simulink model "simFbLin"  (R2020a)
settings: Solver=ode15s  StartTime=0.0  StopTime=tsim  MaxStep=1  RelTol=1e-3
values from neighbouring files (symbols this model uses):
  dQ2 = Q20+0    (= 836)    [runTransformations.m]
  dT0 = T00+0    (= 10)    [runTransformations.m]
  dv2 = v20+0    (= 0)    [runTransformations.m]    (also in FcOL.m = -0.391; runTransfOL.m = -1)
  nd = 2    [runTransformations.m]    (also in Main.m = size(d0,2); Main_OL.m = size(d0,2); runTestCalcBlk.m = size(d0,2); runTransf.m = size(d0,2))
  np = length(p)    [runTransformations.m]    (also in runH2Psim.m = length(param); Main.m = size(p,2); Main_OL.m = size(p,2); runTestCalcBlk.m = size(p,2))
  nu = 1    [runTransformations.m]    (also in runH2Psim.m = length(u0); Main.m; Main_OL.m; runTestCalcBlk.m)
  nx = 2    [runTransformations.m]    (also in H2P_Turbine_driven.m = param(end); runTD.m = length(x0); H2P_Boiler_driven.m = param(end); runBD.m = length(x0))
  p = [p;tau01;tau02]    [runTransformations.m]    (also in Main.m = [N, Fc0, rhoc, rhoh,U,A,cpc,cph]; Main_OL.m = [N, Fc0, rhoc, rhoh,U,A,cpc,cph]; runTestCalcBlk.m = [N, Fc0, rhoc, rhoh,U,A,cpc,cph]; NonlinearMap.m = [U;A;Fc(i);Fh;cpc;cph;Tcin;Thin])
  Q20 = -F*cp*(T10-T20)    (= 836)    [runTransformations.m]
  T00 = 10    [runTransformations.m]
  tdQ2 = 10    [runTransformations.m]
  tdT0 = 10    [runTransformations.m]
  tsp = 10    [runTransformations.m]
  v20 = 0    [runTransformations.m]    (also in runTransfOL.m = v00)
  x0 = [T10;T20]    [runTransformations.m]    (also in runTD.m = [TE0;TD0;TSh0;MD0; MSh0;w0;TA0;0;0;0;0;0;0;0;0;0]; runBD.m = [TE0;TD0;TSh0;MD0; MSh0;w0;TA0;0;0;0;0;0;0;0;0;0]; runFP.m = [TE0;TD0;TSh0;MD0; MSh0;w0;TA0;0;0;0;0;0;0;0]; runFPV2.m = [TE0;TD0;TSh0;MD0; MSh0;w0;TA0;0;0;0;0;0;0;0])
undefined symbols (not defined in the file or in its folder): TanksODE

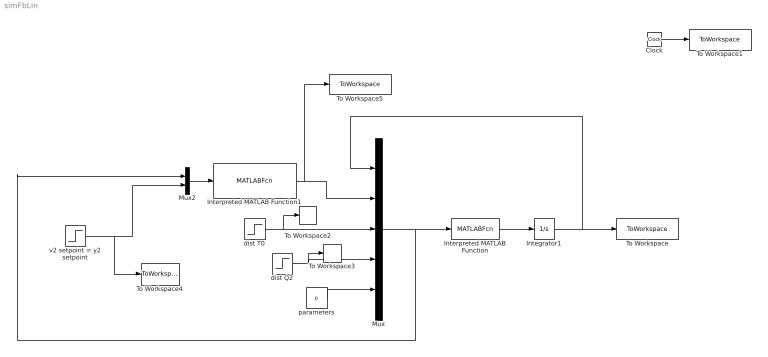
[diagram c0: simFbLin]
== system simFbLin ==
  Clock : Clock
  Integrator1 : Integrator  InitialCondition=x0
  Interpreted MATLAB Function : MATLABFcn  MATLABFcn=TanksODE(u(1:nx),u(nx+1:nx+nu), u(nx+nu+1:nx+nu+nd), u(nx+nu+nd+1:nx+nu+nd+np))
  Interpreted MATLAB Function1 : MATLABFcn  MATLABFcn=FbLin(u(1:nx),u(nx+1:nx+nu), u(nx+nu+1:nx+nu+nd), u(nx+nu+nd+1:nx+nu+nd+np),u(end))
  Mux : Mux  Inputs=5
  Mux2 : Mux  Inputs=2
  To Workspace : ToWorkspace  VariableName=y  SampleTime=-1
  To Workspace1 : ToWorkspace  VariableName=time  SampleTime=-1
  To Workspace2 : ToWorkspace  VariableName=T0  SampleTime=-1
  To Workspace3 : ToWorkspace  VariableName=Q2  SampleTime=-1
  To Workspace4 : ToWorkspace  VariableName=v2  SampleTime=-1
  To Workspace5 : ToWorkspace  VariableName=Q1  SampleTime=-1
  dist Q2 : Step  Time=tdQ2  Before=Q20  After=dQ2  SampleTime=0
  dist T0 : Step  Time=tdT0  Before=T00  After=dT0  SampleTime=0
  parameters : Constant  Value=p
  v2 setpoint = y2 setpoint : Step  Time=tsp  Before=v20  After=dv2  SampleTime=0
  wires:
  Interpreted MATLAB Function/1 -> Integrator1/1
  Mux/1 -> Mux2/1, Interpreted MATLAB Function/1
  parameters/1 -> Mux/5
  dist Q2/1 -> Mux/4, To Workspace3/1
  dist T0/1 -> To Workspace2/1, Mux/3
  Clock/1 -> To Workspace1/1
  v2 setpoint = y2 setpoint/1 -> To Workspace4/1, Mux2/2
  Integrator1/1 -> To Workspace/1, Mux/1
  Interpreted MATLAB Function1/1 -> To Workspace5/1, Mux/2
  Mux2/1 -> Interpreted MATLAB Function1/1
